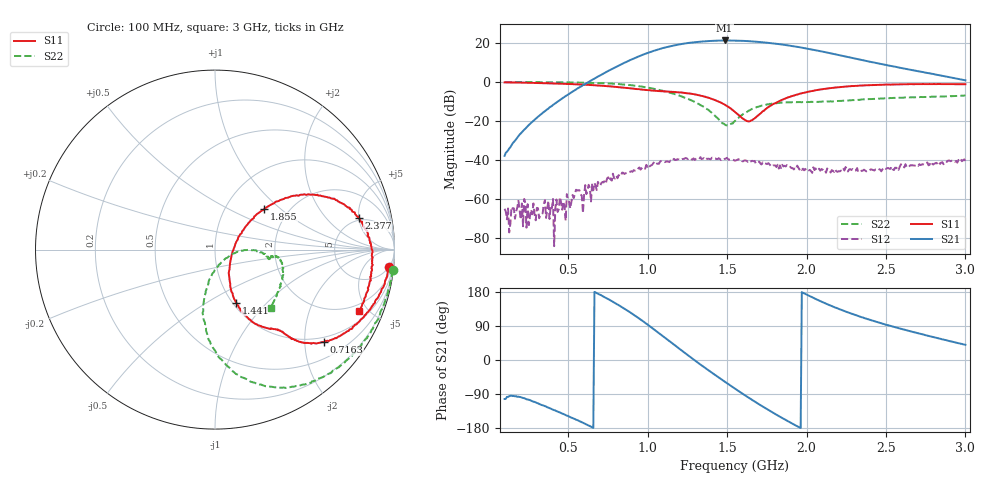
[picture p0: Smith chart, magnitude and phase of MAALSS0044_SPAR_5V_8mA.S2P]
!Part No: MAALSS0044
!Bias: Vdd=5V, Idd=8mA (R1=open)
!2-port de-embedded S-parameters
!Date: Wed Sep 14 16:44:17 2011
!Temp: +25c
!REF Task A17L_2309
!Fixture: 25050XX Rev00
!Test System: Agilent Technologies,E5071C,MY46106711,A.09.61
!Data & Calibration Information:
!Freq	S11:SOLT2(ON)	S21:SOLT2(ON)	S12:SOLT2(ON)	S22:SOLT2(ON)
!PortZ  Port1:50+j0  Port2:50+j0
# Hz S dB R 50
!Freq(Hz)	S11(dB) 	S11(Angle)	S21(dB) 	S21(Angle)	S12(dB) 	S12(Angle)	S22(dB) 	S22(Angle)
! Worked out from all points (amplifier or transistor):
!   401 points, 100 MHz to 3 GHz, reference 50 ohm
!   highest |S21| = 21.3 dB at 1.485 GHz (marker M1)
!   |S21| within 3 dB of that: 1.142 GHz to 1.92 GHz (778.2 MHz wide, 50.8 % of centre)
!   unconditionally stable (mu >= 1): start of sweep to end of sweep
!   at 578.5 MHz: K = 9.74, MAG = 14.7 dB, |S12| = -57.5 dB
!   at 1.55 GHz: K = 4.40, MAG = 21.4 dB, |S12| = -40.4 dB
!   at 3 GHz: K = 8.96, MAG = 8.1 dB, |S12| = -40.5 dB
!   S11 on the Smith chart (normalised r, x): 100 MHz: 5, -19; 716.2 MHz: 0.87, -2.46; 1.441 GHz: 1.04, -0.68; 1.855 GHz: 1.51, +0.79; 2.377 GHz: 4.63, +4.96; 3 GHz: 1.53, -4.40
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1e8  -0.24 -5.7  -37.93 -102.9  -65.06 141.2  -0.03 -6.5
5.8575e8  -1.36 -33.2  -2.08 -164.2  -58.44 144.4  -0.35 -39.4
7.1625e8  -1.97 -40.3  4.05 168.6  -51.32 148.7  -0.66 -50.4
9.1925e8  -3.57 -48.7  12.22 117.5  -45.52 134.4  -1.89 -70.3
9.9175e8  -4.12 -50.1  14.65 95.9  -42.53 128.5  -2.78 -78.1
1.0715e9  -4.70 -51.1  16.78 71.2  -41.99 111.1  -4.09 -85.9
1.173e9  -5.18 -53.6  18.83 38.5  -40.04 90.3  -6.28 -94.8
1.28175e9  -6.17 -59.6  20.25 3.6  -39.84 67.2  -9.70 -101.4
1.3615e9  -7.58 -64.6  20.84 -20.7  -39.69 51.1  -13.23 -102.1
1.44125e9  -9.94 -68.1  21.17 -44.3  -39.54 31.7  -18.72 -91.2
1.48475e9  -11.62 -68.0  21.28 -57.1  -39.50 26.5  -21.79 -66.9
1.55e9  -15.35 -62.4  21.24 -75.6  -40.40 16.4  -20.06 -14.3
1.62975e9  -20.14 -20.7  20.95 -97.8  -40.94 -4.3  -15.15 -0.8
1.71675e9  -15.73 31.2  20.39 -120.8  -42.34 -27.1  -12.14 -2.3
1.782e9  -11.83 39.2  19.83 -137.3  -43.44 -37.4  -11.10 -4.9
1.8545e9  -8.93 39.7  19.11 -154.8  -43.36 -56.9  -10.48 -8.2
1.9415e9  -6.43 36.3  17.99 -174.8  -42.94 -78.2  -10.35 -10.2
2.03575e9  -4.67 31.9  16.62 165.7  -46.62 -100.9  -10.21 -9.6
2.18075e9  -2.89 23.3  14.15 138.4  -44.92 -126.4  -9.80 -7.4
2.3765e9  -1.73 12.4  10.78 109.0  -45.88 -166.2  -8.87 -8.0
2.5215e9  -1.34 5.4  8.34 90.6  -44.49 -163.3  -8.35 -12.9
3e9  -1.18 -23.1  0.83 40.1  -40.47 -173.8  -6.98 -46.1
